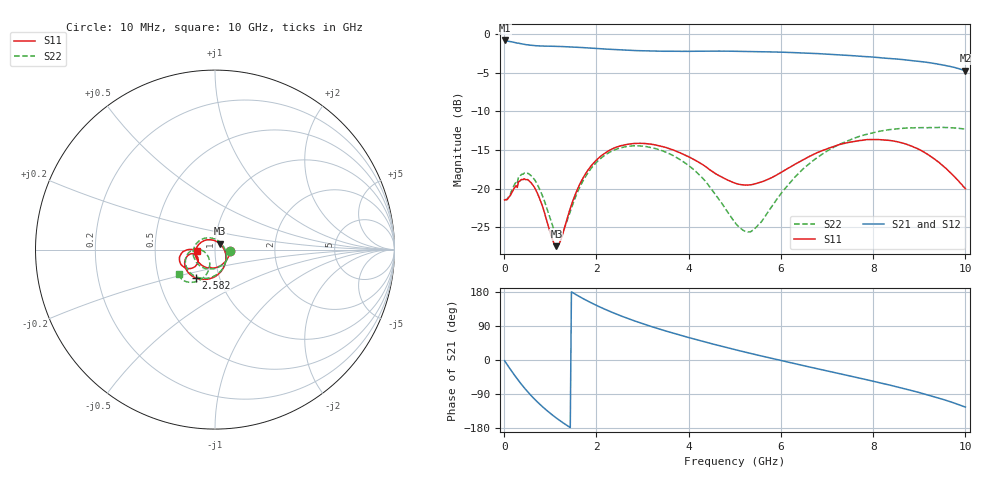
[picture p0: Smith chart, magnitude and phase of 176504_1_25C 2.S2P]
!  2-Port S-parameters saved by WinCal
! VAR MeasName=S-Parameters (CALIBRATED_DATA) read from VNA (N5242A)
! VAR MeasDate=2017-11-2 16:03:10
! VAR NAME=176504_1_25C 2
! VAR FILENAME=176504_1_25C 2.S2P
! VAR DATE=2017-11-2 16:03:10
! VAR PHYS_PORTS=2,3
# Hz S DB R 50
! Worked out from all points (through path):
!   401 points, 10 MHz to 10 GHz, reference 50 ohm
!   highest |S21| = -0.84 dB at 10 MHz (marker M1); lowest = -4.8 dB at 10 GHz (marker M2)
!   lowest |S11| = -27.4 dB at 1.134 GHz (marker M3), VSWR 1.09, Z = 52.7 + j3.4 ohm
!   |S11| at or under -10 dB: start of sweep to end of sweep
!   |S22| runs from -26.2 to -12.1 dB; largest |S21 - S12| = 0.0073
!   S11 on the Smith chart (normalised r, x): 10 MHz: 1.18, -0.02; 2.582 GHz: 0.77, -0.25; 10 GHz: 0.82, -0.01
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1e7  -21.47 -4.7  -0.84 -2.0  -0.84 -2.0  -21.46 -4.7
1.34875e8  -20.89 -58.7  -1.00 -24.6  -1.00 -24.6  -20.69 -61.3
2.5975e8  -19.61 -99.6  -1.14 -45.9  -1.15 -45.9  -19.12 -102.5
3.5965e8  -18.88 -125.5  -1.25 -61.9  -1.26 -61.9  -18.25 -128.3
4.84525e8  -18.84 -153.8  -1.39 -80.3  -1.40 -80.3  -18.04 -156.3
6.34375e8  -19.63 177.0  -1.49 -100.2  -1.50 -100.2  -18.66 174.9
8.092e8  -21.94 143.4  -1.56 -120.8  -1.56 -120.8  -20.61 142.1
1.133875e9  -27.43 49.3  -1.61 -153.4  -1.60 -153.4  -25.94 59.4
1.283725e9  -25.57 -2.7  -1.64 -166.4  -1.64 -166.3  -25.46 8.2
1.683325e9  -18.92 -66.1  -1.76 163.9  -1.76 163.9  -19.29 -63.9
2.1079e9  -15.74 -99.0  -1.92 138.1  -1.92 138.0  -16.02 -99.5
2.582425e9  -14.37 -124.2  -2.08 114.1  -2.08 114.1  -14.64 -126.5
3.35665e9  -14.45 -152.2  -2.23 82.0  -2.25 82.1  -14.96 -157.7
4.2058e9  -16.53 -168.8  -2.23 52.5  -2.24 52.6  -18.07 -179.1
5.005e9  -19.29 -162.3  -2.24 27.4  -2.24 27.4  -24.36 -168.6
5.4046e9  -19.44 -151.7  -2.27 15.5  -2.28 15.6  -25.34 -134.6
6.05395e9  -17.73 -140.5  -2.37 -2.8  -2.38 -2.8  -20.26 -107.9
6.678325e9  -15.65 -141.0  -2.51 -20.0  -2.53 -20.0  -16.46 -109.6
7.577425e9  -13.92 -152.3  -2.83 -44.4  -2.85 -44.3  -13.51 -121.6
8.35165e9  -13.77 -165.5  -3.17 -66.0  -3.22 -66.0  -12.37 -132.2
9.25075e9  -15.83 -178.8  -3.75 -94.4  -3.76 -94.1  -12.11 -140.8
1e10  -20.01 -175.7  -4.76 -124.2  -4.78 -123.9  -12.30 -146.5
